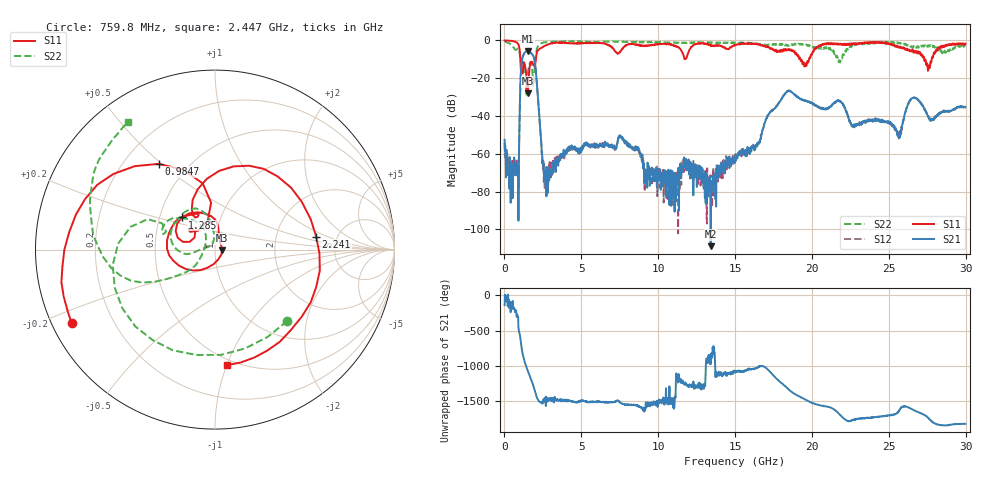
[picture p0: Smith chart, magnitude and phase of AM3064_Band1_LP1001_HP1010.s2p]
# Hz S DB R 50.0
!freq dBS11 angS11 dBS21 angS21 dBS12 angS12 dBS22 angS22
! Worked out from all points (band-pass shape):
!   1600 points, 10 MHz to 29.98 GHz, reference 50 ohm
!   highest |S21| = -5.58 dB at 1.51 GHz (marker M1); lowest = -108.9 dB at 13.41 GHz (marker M2)
!   |S21| within 3 dB of the highest: 1.189 GHz to 1.889 GHz (699.9 MHz wide, 45.5 % of centre)
!   lowest |S11| = -27.9 dB at 1.51 GHz (marker M3), VSWR 1.08, Z = 54.2 - j0.39 ohm
!   |S11| at or under -10 dB: 1.031 GHz to 2.039 GHz (1.008 GHz wide, 65.7 % of centre); 19.25 GHz to 19.81 GHz (555.9 MHz wide, 2.85 % of centre); 27.3 GHz to 27.79 GHz (488.1 MHz wide, 1.77 % of centre)
!   |S22| runs from -29.4 to -0.3 dB; largest |S21 - S12| = 0.007
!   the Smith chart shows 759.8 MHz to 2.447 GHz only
!   S11 on the Smith chart (normalised r, x): 759.8 MHz: 0.06, -0.24; 984.7 MHz: 0.34, +0.49; 1.285 GHz: 0.65, +0.25; 2.241 GHz: 3.46, +0.74; 2.447 GHz: 0.45, -1.00
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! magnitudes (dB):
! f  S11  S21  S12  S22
! 10 MHz  0.0  -52.6  -53.9  -0.3
! 759.8 MHz  -0.9  -71.3  -71.4  -5.0
! 984.7 MHz  -4.9  -41.0  -40.8  -6.2
! 1.135 GHz  -15.1  -10.8  -10.7  -10.7
! 1.285 GHz  -11.8  -7.0  -6.9  -11.9
! 1.51 GHz  -27.9  -5.6  -5.5  -18.2
! 1.922 GHz  -13.2  -9.4  -9.4  -19.0
! 2.241 GHz  -4.9  -37.3  -37.5  -2.3
! 2.447 GHz  -3.8  -59.0  -59.5  -1.3
! 2.822 GHz  -2.2  -69.5  -69.5  -0.9
! 5.015 GHz  -1.5  -57.3  -57.2  -0.7
! 7.582 GHz  -5.5  -51.0  -50.9  -0.5
! 10 GHz  -2.0  -74.5  -70.5  -0.9
! 13.41 GHz  -3.0  -108.9  -71.3  -1.2
! 15 GHz  -2.5  -63.2  -60.4  -1.4
! 18.38 GHz  -4.9  -27.0  -27.0  -2.8
! 19.99 GHz  -7.6  -33.3  -33.2  -3.1
! 25 GHz  -1.5  -43.6  -43.9  -1.0
! 25.69 GHz  -3.6  -49.3  -50.3  -1.5
! 26.61 GHz  -6.5  -30.4  -30.2  -3.0
! 27.56 GHz  -15.8  -40.6  -40.3  -2.6
! 29.98 GHz  -1.8  -35.3  -35.3  -3.1
